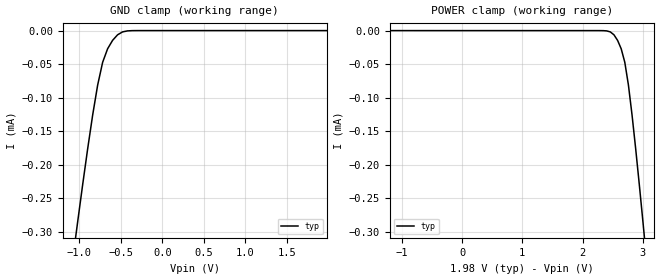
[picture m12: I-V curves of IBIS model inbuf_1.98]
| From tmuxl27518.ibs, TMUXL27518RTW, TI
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| inbuf_1.98
[Model]   inbuf_1.98
Model_type   Input
Vinl = 0.39
Vinh = 0.77
|   typ   min   max
C_comp   2.533030e-13   NA   NA
[Voltage Range]   1.98   NA   NA
[Temperature Range]   27   NA   NA
[Power Clamp Reference]   1.98   NA   NA
[GND Clamp Reference]   0   NA   NA
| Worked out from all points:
|   GND clamp passes 1 mA (typ) near -1.75 V on its own axis
[GND Clamp]
|   Voltage   I(typ)   I(min)   I(max)
-3.96V    -3.277mA   NA         NA
-1.08V    -340.4uA   NA         NA
-1.02V    -284.1uA   NA         NA
-900mV    -175.7uA   NA         NA
-840mV    -125.6uA   NA         NA
-780mV    -81.11uA   NA         NA
-720mV    -47.24uA   NA         NA
-660mV    -27.03uA   NA         NA
-540mV    -6.276uA   NA         NA
-480mV    -1.958uA   NA         NA
-360mV    -77.04nA   NA         NA
1.98V     137.5pA    NA         NA
[POWER Clamp]
|   Voltage   I(typ)   I(min)   I(max)
-1.98V    35.85nA    NA         NA
2.46V     -1.958uA   NA         NA
2.52V     -6.276uA   NA         NA
2.58V     -14.53uA   NA         NA
2.64V     -27.03uA   NA         NA
2.7V      -47.24uA   NA         NA
2.76V     -81.11uA   NA         NA
2.82V     -125.6uA   NA         NA
2.88V     -175.7uA   NA         NA
3V        -284.1uA   NA         NA
3.06V     -340.4uA   NA         NA
3.96V     -1.237mA   NA         NA
